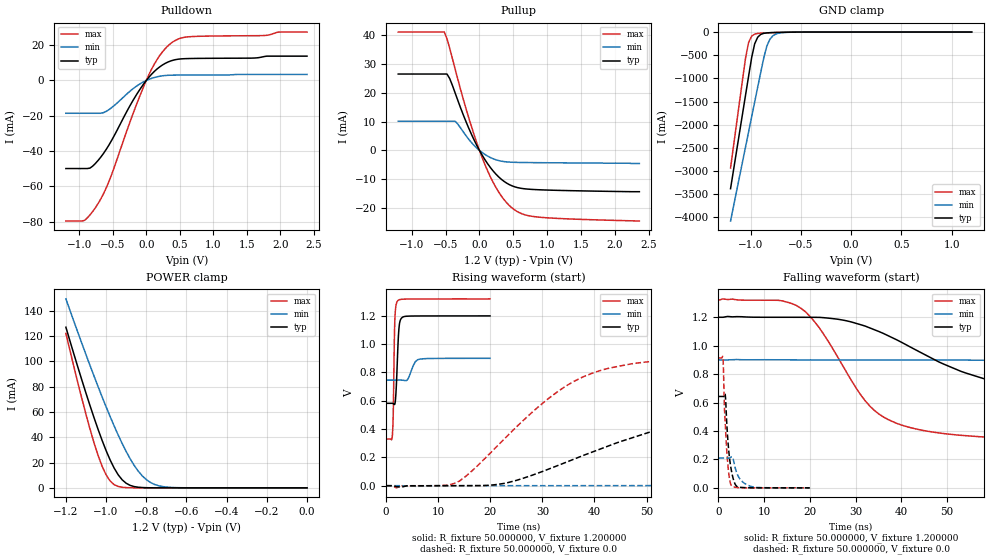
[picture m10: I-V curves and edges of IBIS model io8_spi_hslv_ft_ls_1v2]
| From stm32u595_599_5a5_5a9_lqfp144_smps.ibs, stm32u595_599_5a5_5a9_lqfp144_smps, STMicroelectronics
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|   Model io8_spi_hslv_ft_ls_1v2
[Model]  io8_spi_hslv_ft_ls_1v2
Model_type I/O
Polarity   Non-Inverting
Enable   Active-Low
Vinl =   0.360000V
Vinh =   0.840000V
Vmeas =  0.600000V
Cref =   50.000000pF
Rref =   100.000000M
Vref =   0.0V
C_comp   3.133100pF   3.070300pF   3.178200pF
[Temperature Range]   25.000000   0.140000k   -40.000000
[Pullup Reference]   1.200000V   0.900000V   1.320000V
[Pulldown Reference]   0.0V   0.0V   0.0V
[POWER Clamp Reference]   1.200000V   0.900000V   1.320000V
[GND Clamp Reference]   0.0V   0.0V   0.0V
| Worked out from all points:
|   slope of the pulldown table from 0 to 0.18 V, typ, clamps not added: 25.4 ohm
|   slope of the pullup table from 0 to 0.18 V, typ, clamps not added: 27.8 ohm
|   GND clamp passes 1 mA (typ) near -0.51 V on its own axis
|   POWER clamp passes 1 mA (typ) near -0.86 V on its own axis
|   rising waveform, R_fixture 50.000000, V_fixture 1.200000: 20-80 % time 433ps typ, 1.04ns min, 256ps max; typ from 0.582 V to 1.2 V
|   rising waveform, R_fixture 50.000000, V_fixture 0.0: 20-80 % time 33.6ns typ, 83ns min, 17.1ns max; typ from 0 V to 0.643 V
|   falling waveform, R_fixture 50.000000, V_fixture 1.200000: 20-80 % time 30.3ns typ, 71ns min, 12.6ns max; typ from 1.2 V to 0.582 V
|   falling waveform, R_fixture 50.000000, V_fixture 0.0: 20-80 % time 1.06ns typ, 1.81ns min, 833ps max; typ from 0.643 V to 0 V
[Pulldown]
|Voltage   I(typ)   I(min)   I(max)
-1.2V     -49.85mA   -18.56mA   -79.56mA
-920mV    -49.85mA   -18.56mA   -79.19mA
-840mV    -49.59mA   -18.56mA   -76.08mA
-720mV    -45.32mA   -18.56mA   -69.74mA
-560mV    -36.71mA   -16.57mA   -57.44mA
-200mV    -11.43mA   -4.738mA   -19.03mA
0V        0A         -1.1pA     0A
160mV     6.476mA    2.074mA    11.78mA
360mV     10.99mA    2.987mA    20.81mA
480mV     12.07mA    3.051mA    23.52mA
640mV     12.43mA    3.072mA    24.76mA
2.4V      13.78mA    3.43mA     27.43mA
[Pullup]
|Voltage   I(typ)   I(min)   I(max)
-1.2V     26.53mA    10.15mA    41.1mA
-520mV    26.53mA    10.15mA    41.1mA
-480mV    26.53mA    10.15mA    38.78mA
-440mV    24.95mA    10.15mA    35.49mA
-360mV    19.99mA    10.15mA    28.26mA
-160mV    7.809mA    3.929mA    11.44mA
40mV      -1.649mA   -721.1uA   -2.521mA
240mV     -8.14mA    -3.199mA   -12.72mA
480mV     -12.27mA   -4.076mA   -19.94mA
640mV     -13.22mA   -4.167mA   -22.09mA
880mV     -13.63mA   -4.229mA   -23.14mA
2.36V     -14.3mA    -4.5mA     -24.47mA
[GND_clamp]
|Voltage   I(typ)   I(min)   I(max)
-1.2V     -3.379A    -4.076A    -2.932A
-1.05V    -1.35A     -2.47A     -550.7mA
-1.02V    -947.8mA   -2.149A    -221.5mA
-990mV    -552.4mA   -1.829A    -88.44mA
-960mV    -255.3mA   -1.51A     -44.87mA
-930mV    -111.8mA   -1.191A    -30.68mA
-870mV    -28.35mA   -564.6mA   -21.34mA
-840mV    -18.65mA   -309.5mA   -18.49mA
-810mV    -14.07mA   -161.6mA   -15.92mA
-780mV    -11.37mA   -83.33mA   -13.53mA
-600mV    -3.009mA   -4.321mA   -3.091mA
1.2V      0A         13.65nA    0A
[POWER_clamp]
|Voltage   I(typ)   I(min)   I(max)
-1.2V     127mA      149.4mA    122.2mA
-1.12V    84.97mA    114mA      70.27mA
-1.06V    55.51mA    88.42mA    35.67mA
-1.02V    37.63mA    72.04mA    17.17mA
-1V       29.51mA    64.13mA    10.3mA
-960mV    15.69mA    48.99mA    2.571mA
-900mV    3.624mA    28.77mA    182.8uA
-840mV    490.7uA    13.24mA    11.35uA
-800mV    116.8uA    6.532mA    1.77uA
-740mV    13.2uA     1.723mA    109.1nA
-620mV    167.4nA    79.36uA    0A
0V        0A         17.87nA    0A
[Ramp]
| variable   typ   min   max
dV/dt_r  0.38561/33.59699n   0.12540/82.88731n   0.54825/17.04311n
dV/dt_f  0.37078/30.28387n   92.41200m/70.96060n 0.59435/12.60298n
R_load = 50.000000
[Rising Waveform]
R_fixture= 50.000000
V_fixture= 1.200000
V_fixture_min= 0.900000
V_fixture_max= 1.320000
|time   V(typ)   V(min)   V(max)
0s        582mV      746mV      329.4mV
1.201ns   582mV      746mV      359.1mV
1.361ns   579.9mV    746mV      508.4mV
1.562ns   573.8mV    746mV      1.012V
1.682ns   579.2mV    746mV      1.183V
2.202ns   935.1mV    746.1mV    1.306V
2.563ns   1.145V     746.1mV    1.315V
3.243ns   1.192V     745.2mV    1.318V
6.366ns   1.199V     893.4mV    1.32V
19.94ns   1.2V       900mV      1.32V
[Rising Waveform]
R_fixture= 50.000000
V_fixture= 0.0
V_fixture_min= 0.0
V_fixture_max= 0.0
|time   V(typ)   V(min)   V(max)
0s        1.999nV    239.3nV    1.184nV
13.01ns   -194.8uV   -105.6uV   15.11mV
23.02ns   18.34mV    -70.04uV   342.6mV
36.04ns   187.2mV    140.5uV    736.8mV
43.04ns   285.8mV    307.6uV    832.4mV
57.06ns   447mV      2.531mV    893.9mV
81.08ns   585.9mV    28.06mV    911.6mV
116.1ns   634.5mV    93.54mV    913.7mV
240.2ns   642.7mV    199.9mV    913.7mV
498.5ns   642.7mV    209.2mV    913.8mV
[Falling Waveform]
R_fixture= 50.000000
V_fixture= 1.200000
V_fixture_min= 0.900000
V_fixture_max= 1.320000
|time   V(typ)   V(min)   V(max)
0s        1.2V       900mV      1.32V
17.02ns   1.2V       900.2mV    1.283V
22.02ns   1.199V     900mV      1.126V
31.03ns   1.148V     900mV      656.7mV
35.04ns   1.1V       900mV      520.1mV
43.04ns   971.7mV    900mV      415.2mV
57.06ns   777.5mV    897.9mV    359.6mV
80.08ns   652.8mV    876.6mV    336.1mV
119.1ns   597mV      809.9mV    330.1mV
498.5ns   582mV      746mV      329.4mV
[Falling Waveform]
R_fixture= 50.000000
V_fixture= 0.0
V_fixture_min= 0.0
V_fixture_max= 0.0
|time   V(typ)   V(min)   V(max)
0s        642.7mV    209.2mV    913.8mV
961ps     642.9mV    209.2mV    919.5mV
1.321ns   653.2mV    209.3mV    550.3mV
1.481ns   653.7mV    209.3mV    452.7mV
1.762ns   484.7mV    209.3mV    283.8mV
2.282ns   247.5mV    209.1mV    92.63mV
2.803ns   124.9mV    217.3mV    17.55mV
3.964ns   11.11mV    107.4mV    2.426mV
6.727ns   557.1uV    14.47mV    253.6uV
19.94ns   1.999nV    239.3nV    1.184nV
